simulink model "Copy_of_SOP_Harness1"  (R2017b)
settings: Solver=FixedStepDiscrete  StartTime=0.0  StopTime=17  FixedStep=0.01  RelTol=1e-3  EnableMultiTasking=on
undefined symbols (not defined in the file): sigbuilder_block

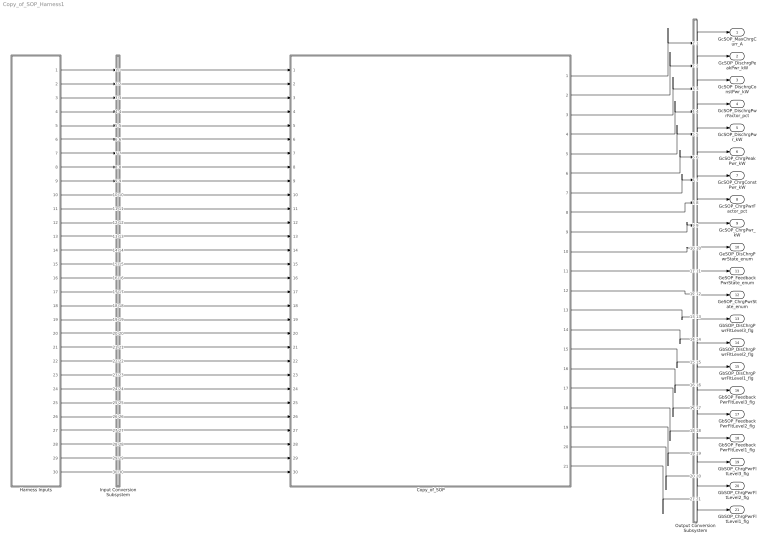
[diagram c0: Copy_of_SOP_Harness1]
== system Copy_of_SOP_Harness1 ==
  Copy_of_SOP : ModelReference  ModelNameDialog=Copy_of_SOP  SimulationMode=Normal  ModelReferenceVersion='M110C115R104'
  Harness Inputs : Subsystem  Tag=STV Subsys  LoadFcn=sigbuilder_block('load');  StartFcn=sigbuilder_block('start');  StopFcn=sigbuilder_block('stop');  ClipboardFcn=sigbuilder_block('clipboard');  mask(Sigbuilder block){tuvar=[0:10]}
      mask init:
      | if ~strcmp(get_param(bdroot(gcb),'SimulationStatus'),'stopped'),tuvar = sigbuilder_block('maskInit'); end
  Input Conversion Subsystem : Subsystem  Tag=__SLT_ICS__  Description=Signal spec. and routing
  Output Conversion Subsystem : Subsystem  Tag=__SLT_OCS__  Description=Signal spec. and routing
  GcSOP_MaxChrgCurr_A : Outport  OutDataTypeStr=single  PortDimensions=[1]
  GcSOP_DischrgPeakPwr_kW : Outport  Port=2  OutDataTypeStr=single  PortDimensions=[1]
  GcSOP_DischrgConstPwr_kW : Outport  Port=3  OutDataTypeStr=single  PortDimensions=[1]
  GcSOP_DischrgPwrFactor_pct : Outport  Port=4  OutDataTypeStr=single  PortDimensions=[1]
  GcSOP_DischrgPwr_kW : Outport  Port=5  OutDataTypeStr=single  PortDimensions=[1]
  GcSOP_ChrgPeakPwr_kW : Outport  Port=6  OutDataTypeStr=single  PortDimensions=[1]
  GcSOP_ChrgConstPwr_kW : Outport  Port=7  OutDataTypeStr=single  PortDimensions=[1]
  GcSOP_ChrgPwrFactor_pct : Outport  Port=8  OutDataTypeStr=single  PortDimensions=[1]
  GcSOP_ChrgPwr_kW : Outport  Port=9  OutDataTypeStr=single  PortDimensions=[1]
  GeSOP_DisChrgPwrState_enum : Outport  Port=10  OutDataTypeStr=uint8  PortDimensions=[1]
  GeSOP_FeedbackPwrState_enum : Outport  Port=11  OutDataTypeStr=uint8  PortDimensions=[1]
  GeSOP_ChrgPwrState_enum : Outport  Port=12  OutDataTypeStr=uint8  PortDimensions=[1]
  GbSOP_DisChrgPwrFltLevel3_flg : Outport  Port=13  OutDataTypeStr=boolean  PortDimensions=[1]
  GbSOP_DisChrgPwrFltLevel2_flg : Outport  Port=14  OutDataTypeStr=boolean  PortDimensions=[1]
  GbSOP_DisChrgPwrFltLevel1_flg : Outport  Port=15  OutDataTypeStr=boolean  PortDimensions=[1]
  GbSOP_FeedbackPwrFltLevel3_flg : Outport  Port=16  OutDataTypeStr=boolean  PortDimensions=[1]
  GbSOP_FeedbackPwrFltLevel2_flg : Outport  Port=17  OutDataTypeStr=boolean  PortDimensions=[1]
  GbSOP_FeedbackPwrFltLevel1_flg : Outport  Port=18  OutDataTypeStr=boolean  PortDimensions=[1]
  GbSOP_ChrgPwrFltLevel3_flg : Outport  Port=19  OutDataTypeStr=boolean  PortDimensions=[1]
  GbSOP_ChrgPwrFltLevel2_flg : Outport  Port=20  OutDataTypeStr=boolean  PortDimensions=[1]
  GbSOP_ChrgPwrFltLevel1_flg : Outport  Port=21  OutDataTypeStr=boolean  PortDimensions=[1]
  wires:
  Harness Inputs/1(GcCDP_MaxCellTemp_C) -> Input Conversion Subsystem/1(Inport_1)
  Harness Inputs/2(GcCDP_MinCellTemp_C) -> Input Conversion Subsystem/2(Inport_2)
  Harness Inputs/3(GcSOC_MaxCellSOC_pct) -> Input Conversion Subsystem/3(Inport_3)
  Harness Inputs/4(GcSOC_MinCellSOC_pct) -> Input Conversion Subsystem/4(Inport_4)
  Harness Inputs/5(GeCTC_CtrCtlConnMode_enum) -> Input Conversion Subsystem/5(Inport_5)
  Harness Inputs/6(GcCDP_MaxCellVolt_mV) -> Input Conversion Subsystem/6(Inport_6)
  Harness Inputs/7(GcCDP_MinCellVolt_mV) -> Input Conversion Subsystem/7(Inport_7)
  Harness Inputs/8(GcHDP_PackVolt_V) -> Input Conversion Subsystem/8(Inport_8)
  Harness Inputs/9(GcCDP_SumCellVolt_V) -> Input Conversion Subsystem/9(Inport_9)
  Harness Inputs/10(GbCDP_SumCellVoltVld_flg) -> Input Conversion Subsystem/10(Inport_10)
  Harness Inputs/11(GeMSM_BMUState_enum) -> Input Conversion Subsystem/11(Inport_11)
  Harness Inputs/12(GcHDP_PackCrnt_A) -> Input Conversion Subsystem/12(Inport_12)
  Harness Inputs/13(GeFTC_FltLevel_enum) -> Input Conversion Subsystem/13(Inport_13)
  Harness Inputs/14(GeCTC_CtrCtlState_enum) -> Input Conversion Subsystem/14(Inport_14)
  Harness Inputs/15(GcACC_ACChrgCrntRqst_A) -> Input Conversion Subsystem/15(Inport_15)
  Harness Inputs/16(GcDCC_DCChrgCrntRqst_A) -> Input Conversion Subsystem/16(Inport_16)
  Harness Inputs/17(GbISP_OpenContactor_flg) -> Input Conversion Subsystem/17(Inport_17)
  Harness Inputs/18(GbISP_PowerDown_flg) -> Input Conversion Subsystem/18(Inport_18)
  Harness Inputs/19(GbISP_DischrgPwrLimitLevel3_flg) -> Input Conversion Subsystem/19(Inport_19)
  Harness Inputs/20(GbISP_RegenPwrLimitLevel3_flg) -> Input Conversion Subsystem/20(Inport_20)
  Harness Inputs/21(GbISP_DischrgPwrLimitLevel2_flg) -> Input Conversion Subsystem/21(Inport_21)
  Harness Inputs/22(GbISP_RegenPwrLimitLevel2_flg) -> Input Conversion Subsystem/22(Inport_22)
  Harness Inputs/23(GbISP_DCChrgCurrLimitLevel2_flg) -> Input Conversion Subsystem/23(Inport_23)
  Harness Inputs/24(GbISP_ACChrgCurrLimitLevel2_flg) -> Input Conversion Subsystem/24(Inport_24)
  Harness Inputs/25(GbISP_DischrgPwrLimitLevel1_flg) -> Input Conversion Subsystem/25(Inport_25)
  Harness Inputs/26(GbISP_RegenPwrLimitLevel1_flg) -> Input Conversion Subsystem/26(Inport_26)
  Harness Inputs/27(GcSOH_PackSOH_pct) -> Input Conversion Subsystem/27(Inport_27)
  Harness Inputs/28(GeUDS_CapSel_enum) -> Input Conversion Subsystem/28(Inport_28)
  Harness Inputs/29(GeUDS_AreaSel_enum) -> Input Conversion Subsystem/29(Inport_29)
  Harness Inputs/30(GbUDS_TestMode1_flg) -> Input Conversion Subsystem/30(Inport_30)
  Output Conversion Subsystem/1(Outport_1) -> GcSOP_MaxChrgCurr_A/1
  Output Conversion Subsystem/2(Outport_2) -> GcSOP_DischrgPeakPwr_kW/1
  Output Conversion Subsystem/3(Outport_3) -> GcSOP_DischrgConstPwr_kW/1
  Output Conversion Subsystem/4(Outport_4) -> GcSOP_DischrgPwrFactor_pct/1
  Output Conversion Subsystem/5(Outport_5) -> GcSOP_DischrgPwr_kW/1
  Output Conversion Subsystem/6(Outport_6) -> GcSOP_ChrgPeakPwr_kW/1
  Output Conversion Subsystem/7(Outport_7) -> GcSOP_ChrgConstPwr_kW/1
  Output Conversion Subsystem/8(Outport_8) -> GcSOP_ChrgPwrFactor_pct/1
  Output Conversion Subsystem/9(Outport_9) -> GcSOP_ChrgPwr_kW/1
  Output Conversion Subsystem/10(Outport_10) -> GeSOP_DisChrgPwrState_enum/1
  Output Conversion Subsystem/11(Outport_11) -> GeSOP_FeedbackPwrState_enum/1
  Output Conversion Subsystem/12(Outport_12) -> GeSOP_ChrgPwrState_enum/1
  Output Conversion Subsystem/13(Outport_13) -> GbSOP_DisChrgPwrFltLevel3_flg/1
  Output Conversion Subsystem/14(Outport_14) -> GbSOP_DisChrgPwrFltLevel2_flg/1
  Output Conversion Subsystem/15(Outport_15) -> GbSOP_DisChrgPwrFltLevel1_flg/1
  Output Conversion Subsystem/16(Outport_16) -> GbSOP_FeedbackPwrFltLevel3_flg/1
  Output Conversion Subsystem/17(Outport_17) -> GbSOP_FeedbackPwrFltLevel2_flg/1
  Output Conversion Subsystem/18(Outport_18) -> GbSOP_FeedbackPwrFltLevel1_flg/1
  Output Conversion Subsystem/19(Outport_19) -> GbSOP_ChrgPwrFltLevel3_flg/1
  Output Conversion Subsystem/20(Outport_20) -> GbSOP_ChrgPwrFltLevel2_flg/1
  Output Conversion Subsystem/21(Outport_21) -> GbSOP_ChrgPwrFltLevel1_flg/1
  Input Conversion Subsystem/1(Outport_1) -> Copy_of_SOP/1
  Input Conversion Subsystem/2(Outport_2) -> Copy_of_SOP/2
  Input Conversion Subsystem/3(Outport_3) -> Copy_of_SOP/3
  Input Conversion Subsystem/4(Outport_4) -> Copy_of_SOP/4
  Input Conversion Subsystem/5(Outport_5) -> Copy_of_SOP/5
  Input Conversion Subsystem/6(Outport_6) -> Copy_of_SOP/6
  Input Conversion Subsystem/7(Outport_7) -> Copy_of_SOP/7
  Input Conversion Subsystem/8(Outport_8) -> Copy_of_SOP/8
  Input Conversion Subsystem/9(Outport_9) -> Copy_of_SOP/9
  Input Conversion Subsystem/10(Outport_10) -> Copy_of_SOP/10
  Input Conversion Subsystem/11(Outport_11) -> Copy_of_SOP/11
  Input Conversion Subsystem/12(Outport_12) -> Copy_of_SOP/12
  Input Conversion Subsystem/13(Outport_13) -> Copy_of_SOP/13
  Input Conversion Subsystem/14(Outport_14) -> Copy_of_SOP/14
  Input Conversion Subsystem/15(Outport_15) -> Copy_of_SOP/15
  Input Conversion Subsystem/16(Outport_16) -> Copy_of_SOP/16
  Input Conversion Subsystem/17(Outport_17) -> Copy_of_SOP/17
  Input Conversion Subsystem/18(Outport_18) -> Copy_of_SOP/18
  Input Conversion Subsystem/19(Outport_19) -> Copy_of_SOP/19
  Input Conversion Subsystem/20(Outport_20) -> Copy_of_SOP/20
  Input Conversion Subsystem/21(Outport_21) -> Copy_of_SOP/21
  Input Conversion Subsystem/22(Outport_22) -> Copy_of_SOP/22
  Input Conversion Subsystem/23(Outport_23) -> Copy_of_SOP/23
  Input Conversion Subsystem/24(Outport_24) -> Copy_of_SOP/24
  Input Conversion Subsystem/25(Outport_25) -> Copy_of_SOP/25
  Input Conversion Subsystem/26(Outport_26) -> Copy_of_SOP/26
  Input Conversion Subsystem/27(Outport_27) -> Copy_of_SOP/27
  Input Conversion Subsystem/28(Outport_28) -> Copy_of_SOP/28
  Input Conversion Subsystem/29(Outport_29) -> Copy_of_SOP/29
  Input Conversion Subsystem/30(Outport_30) -> Copy_of_SOP/30
  Copy_of_SOP/1 -> Output Conversion Subsystem/1(Inport_1)
  Copy_of_SOP/2 -> Output Conversion Subsystem/2(Inport_2)
  Copy_of_SOP/3 -> Output Conversion Subsystem/3(Inport_3)
  Copy_of_SOP/4 -> Output Conversion Subsystem/4(Inport_4)
  Copy_of_SOP/5 -> Output Conversion Subsystem/5(Inport_5)
  Copy_of_SOP/6 -> Output Conversion Subsystem/6(Inport_6)
  Copy_of_SOP/7 -> Output Conversion Subsystem/7(Inport_7)
  Copy_of_SOP/8 -> Output Conversion Subsystem/8(Inport_8)
  Copy_of_SOP/9 -> Output Conversion Subsystem/9(Inport_9)
  Copy_of_SOP/10 -> Output Conversion Subsystem/10(Inport_10)
  Copy_of_SOP/11 -> Output Conversion Subsystem/11(Inport_11)
  Copy_of_SOP/12 -> Output Conversion Subsystem/12(Inport_12)
  Copy_of_SOP/13 -> Output Conversion Subsystem/13(Inport_13)
  Copy_of_SOP/14 -> Output Conversion Subsystem/14(Inport_14)
  Copy_of_SOP/15 -> Output Conversion Subsystem/15(Inport_15)
  Copy_of_SOP/16 -> Output Conversion Subsystem/16(Inport_16)
  Copy_of_SOP/17 -> Output Conversion Subsystem/17(Inport_17)
  Copy_of_SOP/18 -> Output Conversion Subsystem/18(Inport_18)
  Copy_of_SOP/19 -> Output Conversion Subsystem/19(Inport_19)
  Copy_of_SOP/20 -> Output Conversion Subsystem/20(Inport_20)
  Copy_of_SOP/21 -> Output Conversion Subsystem/21(Inport_21)

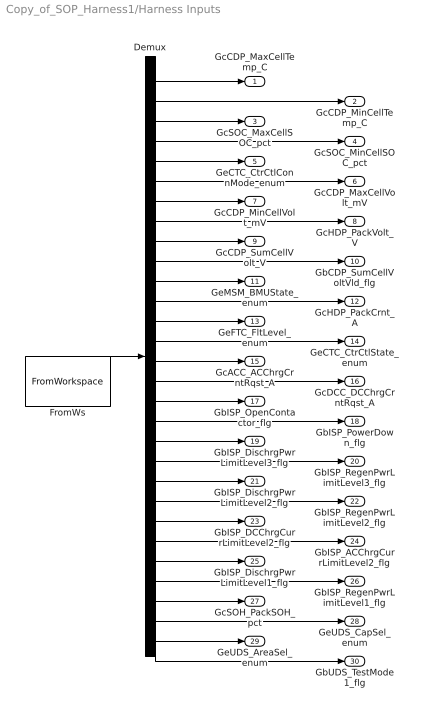
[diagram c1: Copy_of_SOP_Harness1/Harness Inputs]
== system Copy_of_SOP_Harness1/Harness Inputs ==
  Demux : Demux  Tag=STV Demux  Outputs=30
  FromWs : FromWorkspace  Tag=STV FromWs  VariableName=tuvar  SampleTime=0
  GcCDP_MaxCellTemp_C : Outport  Tag=STV Outport
  GcCDP_MinCellTemp_C : Outport  Tag=STV Outport  Port=2
  GcSOC_MaxCellSOC_pct : Outport  Tag=STV Outport  Port=3
  GcSOC_MinCellSOC_pct : Outport  Tag=STV Outport  Port=4
  GeCTC_CtrCtlConnMode_enum : Outport  Tag=STV Outport  Port=5
  GcCDP_MaxCellVolt_mV : Outport  Tag=STV Outport  Port=6
  GcCDP_MinCellVolt_mV : Outport  Tag=STV Outport  Port=7
  GcHDP_PackVolt_V : Outport  Tag=STV Outport  Port=8
  GcCDP_SumCellVolt_V : Outport  Tag=STV Outport  Port=9
  GbCDP_SumCellVoltVld_flg : Outport  Tag=STV Outport  Port=10
  GeMSM_BMUState_enum : Outport  Tag=STV Outport  Port=11
  GcHDP_PackCrnt_A : Outport  Tag=STV Outport  Port=12
  GeFTC_FltLevel_enum : Outport  Tag=STV Outport  Port=13
  GeCTC_CtrCtlState_enum : Outport  Tag=STV Outport  Port=14
  GcACC_ACChrgCrntRqst_A : Outport  Tag=STV Outport  Port=15
  GcDCC_DCChrgCrntRqst_A : Outport  Tag=STV Outport  Port=16
  GbISP_OpenContactor_flg : Outport  Tag=STV Outport  Port=17
  GbISP_PowerDown_flg : Outport  Tag=STV Outport  Port=18
  GbISP_DischrgPwrLimitLevel3_flg : Outport  Tag=STV Outport  Port=19
  GbISP_RegenPwrLimitLevel3_flg : Outport  Tag=STV Outport  Port=20
  GbISP_DischrgPwrLimitLevel2_flg : Outport  Tag=STV Outport  Port=21
  GbISP_RegenPwrLimitLevel2_flg : Outport  Tag=STV Outport  Port=22
  GbISP_DCChrgCurrLimitLevel2_flg : Outport  Tag=STV Outport  Port=23
  GbISP_ACChrgCurrLimitLevel2_flg : Outport  Tag=STV Outport  Port=24
  GbISP_DischrgPwrLimitLevel1_flg : Outport  Tag=STV Outport  Port=25
  GbISP_RegenPwrLimitLevel1_flg : Outport  Tag=STV Outport  Port=26
  GcSOH_PackSOH_pct : Outport  Tag=STV Outport  Port=27
  GeUDS_CapSel_enum : Outport  Tag=STV Outport  Port=28
  GeUDS_AreaSel_enum : Outport  Tag=STV Outport  Port=29
  GbUDS_TestMode1_flg : Outport  Tag=STV Outport  Port=30
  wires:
  FromWs/1 -> Demux/1
  Demux/1 -> GcCDP_MaxCellTemp_C/1
  Demux/2 -> GcCDP_MinCellTemp_C/1
  Demux/3 -> GcSOC_MaxCellSOC_pct/1
  Demux/4 -> GcSOC_MinCellSOC_pct/1
  Demux/5 -> GeCTC_CtrCtlConnMode_enum/1
  Demux/6 -> GcCDP_MaxCellVolt_mV/1
  Demux/7 -> GcCDP_MinCellVolt_mV/1
  Demux/8 -> GcHDP_PackVolt_V/1
  Demux/9 -> GcCDP_SumCellVolt_V/1
  Demux/10 -> GbCDP_SumCellVoltVld_flg/1
  Demux/11 -> GeMSM_BMUState_enum/1
  Demux/12 -> GcHDP_PackCrnt_A/1
  Demux/13 -> GeFTC_FltLevel_enum/1
  Demux/14 -> GeCTC_CtrCtlState_enum/1
  Demux/15 -> GcACC_ACChrgCrntRqst_A/1
  Demux/16 -> GcDCC_DCChrgCrntRqst_A/1
  Demux/17 -> GbISP_OpenContactor_flg/1
  Demux/18 -> GbISP_PowerDown_flg/1
  Demux/19 -> GbISP_DischrgPwrLimitLevel3_flg/1
  Demux/20 -> GbISP_RegenPwrLimitLevel3_flg/1
  Demux/21 -> GbISP_DischrgPwrLimitLevel2_flg/1
  Demux/22 -> GbISP_RegenPwrLimitLevel2_flg/1
  Demux/23 -> GbISP_DCChrgCurrLimitLevel2_flg/1
  Demux/24 -> GbISP_ACChrgCurrLimitLevel2_flg/1
  Demux/25 -> GbISP_DischrgPwrLimitLevel1_flg/1
  Demux/26 -> GbISP_RegenPwrLimitLevel1_flg/1
  Demux/27 -> GcSOH_PackSOH_pct/1
  Demux/28 -> GeUDS_CapSel_enum/1
  Demux/29 -> GeUDS_AreaSel_enum/1
  Demux/30 -> GbUDS_TestMode1_flg/1

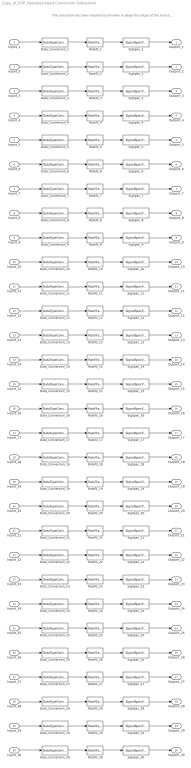
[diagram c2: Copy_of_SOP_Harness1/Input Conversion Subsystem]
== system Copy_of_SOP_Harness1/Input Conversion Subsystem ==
  note: This subsystem has been inserted by Simulink to adapt the output of the source blocks to the interface required by the harnessed component. Modifying the contents of this subsystem may result in compilation and simulation failure.
  Inport_1 : Inport
  Inport_2 : Inport  Port=2
  Inport_3 : Inport  Port=3
  Inport_4 : Inport  Port=4
  Inport_5 : Inport  Port=5
  Inport_6 : Inport  Port=6
  Inport_7 : Inport  Port=7
  Inport_8 : Inport  Port=8
  Inport_9 : Inport  Port=9
  Inport_10 : Inport  Port=10
  Inport_11 : Inport  Port=11
  Inport_12 : Inport  Port=12
  Inport_13 : Inport  Port=13
  Inport_14 : Inport  Port=14
  Inport_15 : Inport  Port=15
  Inport_16 : Inport  Port=16
  Inport_17 : Inport  Port=17
  Inport_18 : Inport  Port=18
  Inport_19 : Inport  Port=19
  Inport_20 : Inport  Port=20
  Inport_21 : Inport  Port=21
  Inport_22 : Inport  Port=22
  Inport_23 : Inport  Port=23
  Inport_24 : Inport  Port=24
  Inport_25 : Inport  Port=25
  Inport_26 : Inport  Port=26
  Inport_27 : Inport  Port=27
  Inport_28 : Inport  Port=28
  Inport_29 : Inport  Port=29
  Inport_30 : Inport  Port=30
  Data_Conversion_{1..4,8..9,12,15..16,27} (10 alike) : DataTypeConversion  OutDataTypeStr=single
  Data_Conversion_{10,17..26,30} (12 alike) : DataTypeConversion  OutDataTypeStr=boolean
  Data_Conversion_{5,11,13..14,28..29} (6 alike) : DataTypeConversion  OutDataTypeStr=uint8
  Data_Conversion_6 : DataTypeConversion  OutDataTypeStr=uint16
  Data_Conversion_7 : DataTypeConversion  OutDataTypeStr=uint16
  RateTs_{1..30} (30 alike) : RateTransition  OutPortSampleTime=0.01
  SigSpec_1 : SignalSpecification  OutDataTypeStr=single  Unit=C  Dimensions=[1]  SampleTime=0.01
  SigSpec_{10,17..26,30} (12 alike) : SignalSpecification  OutDataTypeStr=boolean  Unit=flag  Dimensions=[1]  SampleTime=0.01
  SigSpec_{5,11,13..14,28..29} (6 alike) : SignalSpecification  OutDataTypeStr=uint8  Unit=enum  Dimensions=[1]  SampleTime=0.01
  SigSpec_12 : SignalSpecification  OutDataTypeStr=single  Unit=A  Dimensions=[1]  SampleTime=0.01
  SigSpec_15 : SignalSpecification  OutDataTypeStr=single  Unit=A  Dimensions=[1]  SampleTime=0.01
  SigSpec_16 : SignalSpecification  OutDataTypeStr=single  Unit=A  Dimensions=[1]  SampleTime=0.01
  SigSpec_2 : SignalSpecification  OutDataTypeStr=single  Unit=C  Dimensions=[1]  SampleTime=0.01
  SigSpec_27 : SignalSpecification  OutDataTypeStr=single  Unit=pct  Dimensions=[1]  SampleTime=0.01
  SigSpec_3 : SignalSpecification  OutDataTypeStr=single  Unit=pct  Dimensions=[1]  SampleTime=0.01
  SigSpec_4 : SignalSpecification  OutDataTypeStr=single  Unit=pct  Dimensions=[1]  SampleTime=0.01
  SigSpec_6 : SignalSpecification  OutDataTypeStr=uint16  Unit=mV  Dimensions=[1]  SampleTime=0.01
  SigSpec_7 : SignalSpecification  OutDataTypeStr=uint16  Unit=mV  Dimensions=[1]  SampleTime=0.01
  SigSpec_8 : SignalSpecification  OutDataTypeStr=single  Unit=V  Dimensions=[1]  SampleTime=0.01
  SigSpec_9 : SignalSpecification  OutDataTypeStr=single  Unit=V  Dimensions=[1]  SampleTime=0.01
  Outport_1 : Outport
  Outport_2 : Outport  Port=2
  Outport_3 : Outport  Port=3
  Outport_4 : Outport  Port=4
  Outport_5 : Outport  Port=5
  Outport_6 : Outport  Port=6
  Outport_7 : Outport  Port=7
  Outport_8 : Outport  Port=8
  Outport_9 : Outport  Port=9
  Outport_10 : Outport  Port=10
  Outport_11 : Outport  Port=11
  Outport_12 : Outport  Port=12
  Outport_13 : Outport  Port=13
  Outport_14 : Outport  Port=14
  Outport_15 : Outport  Port=15
  Outport_16 : Outport  Port=16
  Outport_17 : Outport  Port=17
  Outport_18 : Outport  Port=18
  Outport_19 : Outport  Port=19
  Outport_20 : Outport  Port=20
  Outport_21 : Outport  Port=21
  Outport_22 : Outport  Port=22
  Outport_23 : Outport  Port=23
  Outport_24 : Outport  Port=24
  Outport_25 : Outport  Port=25
  Outport_26 : Outport  Port=26
  Outport_27 : Outport  Port=27
  Outport_28 : Outport  Port=28
  Outport_29 : Outport  Port=29
  Outport_30 : Outport  Port=30
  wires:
  SigSpec_1/1 -> Outport_1/1
  RateTs_1/1 -> SigSpec_1/1
  Data_Conversion_1/1 -> RateTs_1/1
  Inport_1/1 -> Data_Conversion_1/1
  SigSpec_2/1 -> Outport_2/1
  RateTs_2/1 -> SigSpec_2/1
  Data_Conversion_2/1 -> RateTs_2/1
  Inport_2/1 -> Data_Conversion_2/1
  SigSpec_3/1 -> Outport_3/1
  RateTs_3/1 -> SigSpec_3/1
  Data_Conversion_3/1 -> RateTs_3/1
  Inport_3/1 -> Data_Conversion_3/1
  SigSpec_4/1 -> Outport_4/1
  RateTs_4/1 -> SigSpec_4/1
  Data_Conversion_4/1 -> RateTs_4/1
  Inport_4/1 -> Data_Conversion_4/1
  SigSpec_5/1 -> Outport_5/1
  RateTs_5/1 -> SigSpec_5/1
  Data_Conversion_5/1 -> RateTs_5/1
  Inport_5/1 -> Data_Conversion_5/1
  SigSpec_6/1 -> Outport_6/1
  RateTs_6/1 -> SigSpec_6/1
  Data_Conversion_6/1 -> RateTs_6/1
  Inport_6/1 -> Data_Conversion_6/1
  SigSpec_7/1 -> Outport_7/1
  RateTs_7/1 -> SigSpec_7/1
  Data_Conversion_7/1 -> RateTs_7/1
  Inport_7/1 -> Data_Conversion_7/1
  SigSpec_8/1 -> Outport_8/1
  RateTs_8/1 -> SigSpec_8/1
  Data_Conversion_8/1 -> RateTs_8/1
  Inport_8/1 -> Data_Conversion_8/1
  SigSpec_9/1 -> Outport_9/1
  RateTs_9/1 -> SigSpec_9/1
  Data_Conversion_9/1 -> RateTs_9/1
  Inport_9/1 -> Data_Conversion_9/1
  SigSpec_10/1 -> Outport_10/1
  RateTs_10/1 -> SigSpec_10/1
  Data_Conversion_10/1 -> RateTs_10/1
  Inport_10/1 -> Data_Conversion_10/1
  SigSpec_11/1 -> Outport_11/1
  RateTs_11/1 -> SigSpec_11/1
  Data_Conversion_11/1 -> RateTs_11/1
  Inport_11/1 -> Data_Conversion_11/1
  SigSpec_12/1 -> Outport_12/1
  RateTs_12/1 -> SigSpec_12/1
  Data_Conversion_12/1 -> RateTs_12/1
  Inport_12/1 -> Data_Conversion_12/1
  SigSpec_13/1 -> Outport_13/1
  RateTs_13/1 -> SigSpec_13/1
  Data_Conversion_13/1 -> RateTs_13/1
  Inport_13/1 -> Data_Conversion_13/1
  SigSpec_14/1 -> Outport_14/1
  RateTs_14/1 -> SigSpec_14/1
  Data_Conversion_14/1 -> RateTs_14/1
  Inport_14/1 -> Data_Conversion_14/1
  SigSpec_15/1 -> Outport_15/1
  RateTs_15/1 -> SigSpec_15/1
  Data_Conversion_15/1 -> RateTs_15/1
  Inport_15/1 -> Data_Conversion_15/1
  SigSpec_16/1 -> Outport_16/1
  RateTs_16/1 -> SigSpec_16/1
  Data_Conversion_16/1 -> RateTs_16/1
  Inport_16/1 -> Data_Conversion_16/1
  SigSpec_17/1 -> Outport_17/1
  RateTs_17/1 -> SigSpec_17/1
  Data_Conversion_17/1 -> RateTs_17/1
  Inport_17/1 -> Data_Conversion_17/1
  SigSpec_18/1 -> Outport_18/1
  RateTs_18/1 -> SigSpec_18/1
  Data_Conversion_18/1 -> RateTs_18/1
  Inport_18/1 -> Data_Conversion_18/1
  SigSpec_19/1 -> Outport_19/1
  RateTs_19/1 -> SigSpec_19/1
  Data_Conversion_19/1 -> RateTs_19/1
  Inport_19/1 -> Data_Conversion_19/1
  SigSpec_20/1 -> Outport_20/1
  RateTs_20/1 -> SigSpec_20/1
  Data_Conversion_20/1 -> RateTs_20/1
  Inport_20/1 -> Data_Conversion_20/1
  SigSpec_21/1 -> Outport_21/1
  RateTs_21/1 -> SigSpec_21/1
  Data_Conversion_21/1 -> RateTs_21/1
  Inport_21/1 -> Data_Conversion_21/1
  SigSpec_22/1 -> Outport_22/1
  RateTs_22/1 -> SigSpec_22/1
  Data_Conversion_22/1 -> RateTs_22/1
  Inport_22/1 -> Data_Conversion_22/1
  SigSpec_23/1 -> Outport_23/1
  RateTs_23/1 -> SigSpec_23/1
  Data_Conversion_23/1 -> RateTs_23/1
  Inport_23/1 -> Data_Conversion_23/1
  SigSpec_24/1 -> Outport_24/1
  RateTs_24/1 -> SigSpec_24/1
  Data_Conversion_24/1 -> RateTs_24/1
  Inport_24/1 -> Data_Conversion_24/1
  SigSpec_25/1 -> Outport_25/1
  RateTs_25/1 -> SigSpec_25/1
  Data_Conversion_25/1 -> RateTs_25/1
  Inport_25/1 -> Data_Conversion_25/1
  SigSpec_26/1 -> Outport_26/1
  RateTs_26/1 -> SigSpec_26/1
  Data_Conversion_26/1 -> RateTs_26/1
  Inport_26/1 -> Data_Conversion_26/1
  SigSpec_27/1 -> Outport_27/1
  RateTs_27/1 -> SigSpec_27/1
  Data_Conversion_27/1 -> RateTs_27/1
  Inport_27/1 -> Data_Conversion_27/1
  SigSpec_28/1 -> Outport_28/1
  RateTs_28/1 -> SigSpec_28/1
  Data_Conversion_28/1 -> RateTs_28/1
  Inport_28/1 -> Data_Conversion_28/1
  SigSpec_29/1 -> Outport_29/1
  RateTs_29/1 -> SigSpec_29/1
  Data_Conversion_29/1 -> RateTs_29/1
  Inport_29/1 -> Data_Conversion_29/1
  SigSpec_30/1 -> Outport_30/1
  RateTs_30/1 -> SigSpec_30/1
  Data_Conversion_30/1 -> RateTs_30/1
  Inport_30/1 -> Data_Conversion_30/1

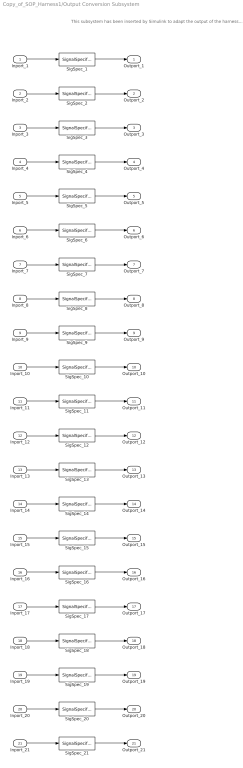
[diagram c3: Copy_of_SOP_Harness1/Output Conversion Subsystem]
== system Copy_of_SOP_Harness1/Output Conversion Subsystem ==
  note: This subsystem has been inserted by Simulink to adapt the output of the harnessed component to the interface required by the sink blocks. Modifying the contents of this subsystem may result in compilation and simulation failure.
  Inport_1 : Inport
  Inport_2 : Inport  Port=2
  Inport_3 : Inport  Port=3
  Inport_4 : Inport  Port=4
  Inport_5 : Inport  Port=5
  Inport_6 : Inport  Port=6
  Inport_7 : Inport  Port=7
  Inport_8 : Inport  Port=8
  Inport_9 : Inport  Port=9
  Inport_10 : Inport  Port=10
  Inport_11 : Inport  Port=11
  Inport_12 : Inport  Port=12
  Inport_13 : Inport  Port=13
  Inport_14 : Inport  Port=14
  Inport_15 : Inport  Port=15
  Inport_16 : Inport  Port=16
  Inport_17 : Inport  Port=17
  Inport_18 : Inport  Port=18
  Inport_19 : Inport  Port=19
  Inport_20 : Inport  Port=20
  Inport_21 : Inport  Port=21
  SigSpec_1 : SignalSpecification  OutDataTypeStr=single  Unit=A  Dimensions=[1]  SampleTime=0.01
  SigSpec_10 : SignalSpecification  OutDataTypeStr=uint8  Unit=enum  Dimensions=[1]  SampleTime=0.01
  SigSpec_11 : SignalSpecification  OutDataTypeStr=uint8  Unit=enum  Dimensions=[1]  SampleTime=0.01
  SigSpec_12 : SignalSpecification  OutDataTypeStr=uint8  Unit=enum  Dimensions=[1]  SampleTime=0.01
  SigSpec_{13..21} (9 alike) : SignalSpecification  OutDataTypeStr=boolean  Unit=flag  Dimensions=[1]  SampleTime=0.01
  SigSpec_{2..3,5..7,9} (6 alike) : SignalSpecification  OutDataTypeStr=single  Unit=kW  Dimensions=[1]  SampleTime=0.01
  SigSpec_4 : SignalSpecification  OutDataTypeStr=single  Unit=pct  Dimensions=[1]  SampleTime=0.01
  SigSpec_8 : SignalSpecification  OutDataTypeStr=single  Unit=pct  Dimensions=[1]  SampleTime=0.01
  Outport_1 : Outport
  Outport_2 : Outport  Port=2
  Outport_3 : Outport  Port=3
  Outport_4 : Outport  Port=4
  Outport_5 : Outport  Port=5
  Outport_6 : Outport  Port=6
  Outport_7 : Outport  Port=7
  Outport_8 : Outport  Port=8
  Outport_9 : Outport  Port=9
  Outport_10 : Outport  Port=10
  Outport_11 : Outport  Port=11
  Outport_12 : Outport  Port=12
  Outport_13 : Outport  Port=13
  Outport_14 : Outport  Port=14
  Outport_15 : Outport  Port=15
  Outport_16 : Outport  Port=16
  Outport_17 : Outport  Port=17
  Outport_18 : Outport  Port=18
  Outport_19 : Outport  Port=19
  Outport_20 : Outport  Port=20
  Outport_21 : Outport  Port=21
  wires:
  Inport_1/1 -> SigSpec_1/1
  SigSpec_1/1 -> Outport_1/1
  Inport_2/1 -> SigSpec_2/1
  SigSpec_2/1 -> Outport_2/1
  Inport_3/1 -> SigSpec_3/1
  SigSpec_3/1 -> Outport_3/1
  Inport_4/1 -> SigSpec_4/1
  SigSpec_4/1 -> Outport_4/1
  Inport_5/1 -> SigSpec_5/1
  SigSpec_5/1 -> Outport_5/1
  Inport_6/1 -> SigSpec_6/1
  SigSpec_6/1 -> Outport_6/1
  Inport_7/1 -> SigSpec_7/1
  SigSpec_7/1 -> Outport_7/1
  Inport_8/1 -> SigSpec_8/1
  SigSpec_8/1 -> Outport_8/1
  Inport_9/1 -> SigSpec_9/1
  SigSpec_9/1 -> Outport_9/1
  Inport_10/1 -> SigSpec_10/1
  SigSpec_10/1 -> Outport_10/1
  Inport_11/1 -> SigSpec_11/1
  SigSpec_11/1 -> Outport_11/1
  Inport_12/1 -> SigSpec_12/1
  SigSpec_12/1 -> Outport_12/1
  Inport_13/1 -> SigSpec_13/1
  SigSpec_13/1 -> Outport_13/1
  Inport_14/1 -> SigSpec_14/1
  SigSpec_14/1 -> Outport_14/1
  Inport_15/1 -> SigSpec_15/1
  SigSpec_15/1 -> Outport_15/1
  Inport_16/1 -> SigSpec_16/1
  SigSpec_16/1 -> Outport_16/1
  Inport_17/1 -> SigSpec_17/1
  SigSpec_17/1 -> Outport_17/1
  Inport_18/1 -> SigSpec_18/1
  SigSpec_18/1 -> Outport_18/1
  Inport_19/1 -> SigSpec_19/1
  SigSpec_19/1 -> Outport_19/1
  Inport_20/1 -> SigSpec_20/1
  SigSpec_20/1 -> Outport_20/1
  Inport_21/1 -> SigSpec_21/1
  SigSpec_21/1 -> Outport_21/1
